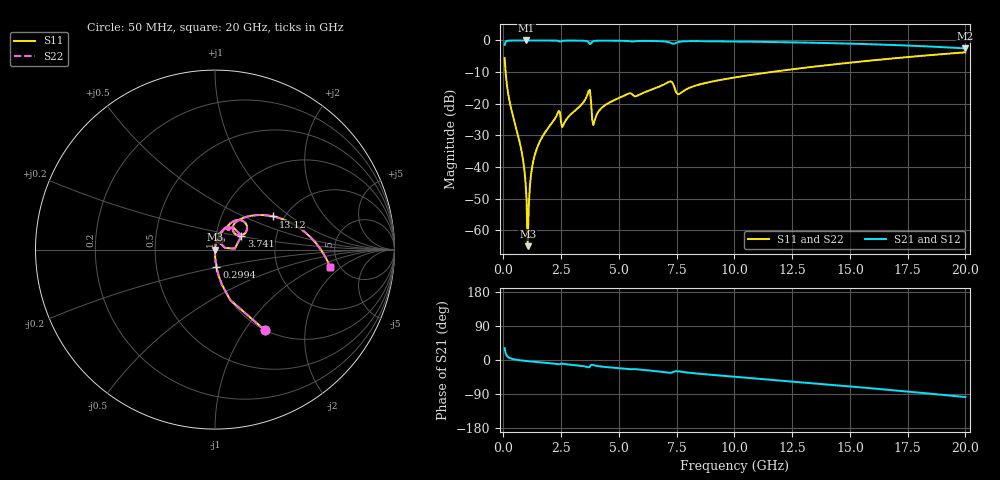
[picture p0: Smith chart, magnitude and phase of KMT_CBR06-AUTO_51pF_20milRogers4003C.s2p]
! Data measured by Modelithics Inc. support@modelithics.com 813-866-6335
! KEMET CBR06-AUTO 51pF, Pad Width= 0.851mm, Pad Length= 0.64mm, Pad Gap= 0.62mm, 20mil Rogers 4003C substrate Data, January 2022
# hz S ma R 50
! 2 Port Network Data from SP1.SP block
! freq  magS11  angS11  magS21  angS21  magS12  angS12  magS22  angS22
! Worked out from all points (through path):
!   401 points, 50 MHz to 20 GHz, reference 50 ohm
!   highest |S21| = 0.00 dB at 997.6 MHz (marker M1); lowest = -2.5 dB at 20 GHz (marker M2)
!   group delay of S21, straight-line fit = 13.7 ps
!   lowest |S11| = -65.0 dB at 1.048 GHz (marker M3), VSWR 1.00, Z = 50 - j0.0349 ohm
!   |S11| at or under -10 dB: 93.79 MHz to 11.57 GHz (11.48 GHz wide, 197 % of centre)
!   |S22| runs from -65.0 to -3.8 dB; largest |S21 - S12| = 0
!   S11 on the Smith chart (normalised r, x): 50 MHz: 1.00, -1.24; 299.4 MHz: 1.00, -0.19; 3.741 GHz: 1.33, +0.21; 13.12 GHz: 1.75, +0.75; 20 GHz: 4.19, -1.43
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5e7  0.5268 -58.3  0.8497 31.6  0.8497 31.6  0.5268 -58.3
2.99375e8  0.09505 -85.3  0.9952 4.6  0.9952 4.6  0.09505 -85.3
7.98125e8  0.01671 -90.0  0.9994 -1.4  0.9994 -1.4  0.01671 -90.0
9.97625e8  0.003273 -84.8  0.9995 -2.7  0.9995 -2.7  0.003273 -84.8
1.0475e9  0.0005645 -38.1  0.9995 -3.1  0.9995 -3.1  0.0005645 -38.1
1.14725e9  0.005168 80.9  0.9995 -3.7  0.9995 -3.7  0.005168 80.9
1.296875e9  0.01268 83.1  0.9993 -4.5  0.9993 -4.5  0.01268 83.1
1.646e9  0.02854 82.2  0.9989 -6.5  0.9989 -6.5  0.02854 82.2
2.34425e9  0.07024 71.4  0.988 -10.9  0.988 -10.9  0.07024 71.4
2.593625e9  0.04607 68.1  0.9895 -10.2  0.9895 -10.2  0.04607 68.1
3.391625e9  0.09807 72.0  0.9909 -15.6  0.9909 -15.6  0.09807 72.0
3.74075e9  0.166 27.7  0.8763 -17.7  0.8763 -17.7  0.166 27.7
3.94025e9  0.05265 56.7  0.9815 -14.4  0.9815 -14.4  0.05265 56.7
4.688375e9  0.1092 68.6  0.9912 -20.0  0.9912 -20.0  0.1092 68.6
6.73325e9  0.1858 57.3  0.9747 -30.3  0.9747 -30.3  0.1858 57.3
7.232e9  0.2252 41.4  0.9176 -33.7  0.9176 -33.7  0.2252 41.4
7.631e9  0.1443 45.5  0.9544 -30.3  0.9544 -30.3  0.1443 45.5
1.0025e10  0.2609 45.1  0.962 -44.2  0.962 -44.2  0.2609 45.1
1.311725e10  0.3732 29.7  0.9242 -59.8  0.9242 -59.8  0.3732 29.7
1.336662e10  0.3825 28.4  0.9203 -61.1  0.9203 -61.1  0.3825 28.4
1.670825e10  0.5139 10.5  0.852 -78.9  0.852 -78.9  0.5139 10.5
2e10  0.6494 -8.7  0.7482 -97.7  0.7482 -97.7  0.6494 -8.7
